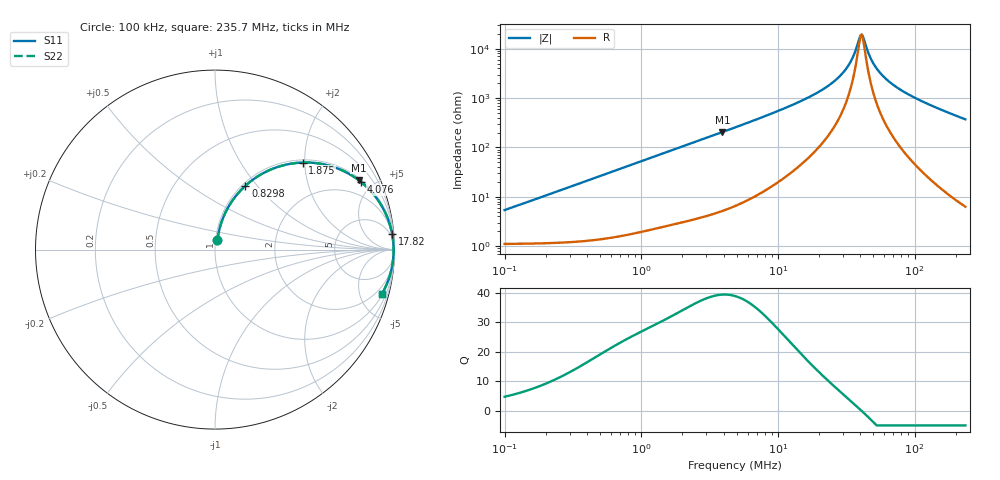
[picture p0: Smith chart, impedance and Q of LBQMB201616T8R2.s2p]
! LBQMB201616T8R2  S-PARAMETER MODEL  ( General Type )
! Model Generated by TAIYO YUDEN Corporation (http://www.ty-top.com)
! Version 1.0
! TAIYO YUDEN Control No. 191025NI43SB-FBB
! Copyright(c) 2019 TAIYO YUDEN CO.,LTD. All Rights Reserved.
! Product Description (link to TY-COMPAS)
! https://ds.yuden.co.jp/TYCOMPAS/or/detail?pn=LBQMB201616T8R2J&u=M
! Products Name : Inductors
! Characteristics :
!  Inductance : 8.2 uH , SRF(min) : 30 MHz , DC Resistance(max) : 1.43 Ohm , Rated Current : 225 mA
!  Case Size : 2.0 x 1.6 / 0.079 x 0.063 [mm/inch] , Thickness : 1.6 / 0.063 [mm/inch]
!  (Conditions: Temperature = 25 degC , DC Bias Current/Voltage = 0A / 0V)
! External Node Assignments :
!  1  o---GGG---o  2
! GND o---------o GND
! Frequency Range : 0.1MHz  -  235.669543MHz  [ 402 STEP ]
# MHz S RI R 50
! Freq[MHz].  S11 Real  S11 Imag  S21 Real  S21 Imag  S12 Real  S12 Imag  S22 Real  S22 Imag
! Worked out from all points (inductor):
!   401 points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, 100 kHz to 235.7 MHz, reference 50 ohm
!   read as one part in series: L = 8.41 uH near 104 kHz
!   highest Q = 39.5 at 3.921 MHz (marker M1), where L = 8.28 uH
!   self-resonance near 40.28 MHz
!   S11 on the Smith chart (normalised r, x): 100 kHz: 1.02, +0.11; 829.8 kHz: 1.03, +0.87; 1.875 MHz: 1.06, +1.95; 4.076 MHz: 1.11, +4.24; 17.82 MHz: 2, +23; 235.7 MHz: 1.13, -7.42
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0.1  0.0137 0.0516  0.9863 -0.0516  0.9863 -0.0516  0.0137 0.0516
0.367165  0.0473 0.1823  0.9527 -0.1823  0.9527 -0.1823  0.0473 0.1823
0.82976  0.1694 0.3556  0.8306 -0.3556  0.8306 -0.3556  0.1694 0.3556
1.348099  0.3365 0.4561  0.6635 -0.4561  0.6635 -0.4561  0.3365 0.4561
1.875187  0.4881 0.4851  0.5119 -0.4851  0.5119 -0.4851  0.4881 0.4851
3.921149  0.8004 0.3872  0.1996 -0.3872  0.1996 -0.3872  0.8004 0.3872
4.076382  0.8123 0.378  0.1877 -0.378  0.1877 -0.378  0.8123 0.378
4.854581  0.8592 0.3352  0.1408 -0.3352  0.1408 -0.3352  0.8592 0.3352
10.15127  0.9628 0.1719  0.0372 -0.1719  0.0372 -0.1719  0.9628 0.1719
17.8243  0.9867 0.0868  0.0133 -0.0868  0.0133 -0.0868  0.9867 0.0868
24.3167  0.9919 0.0511  0.0081 -0.0511  0.0081 -0.0511  0.9919 0.0511
30.10531  0.9938 0.0293  0.00619 -0.0293  0.00619 -0.0293  0.9938 0.0293
34.48723  0.9945 0.0162  0.0055 -0.0162  0.0055 -0.0162  0.9945 0.0162
39.50697  0.9949 0.0033  0.00515 -0.0033  0.00515 -0.0033  0.9949 0.0033
41.07099  0.9949 -0.000367  0.00511 0.000367  0.00511 0.000367  0.9949 -0.000367
42.69694  0.9949 -0.00404  0.0051 0.00404  0.0051 0.00404  0.9949 -0.00404
47.04901  0.9948 -0.0133  0.00518 0.0133  0.00518 0.0133  0.9948 -0.0133
50.84796  0.9946 -0.0207  0.00537 0.0207  0.00537 0.0207  0.9946 -0.0207
57.12919  0.9941 -0.0322  0.00589 0.0322  0.00589 0.0322  0.9941 -0.0322
65.44454  0.9931 -0.0461  0.00687 0.0461  0.00687 0.0461  0.9931 -0.0461
106.3267  0.9846 -0.1043  0.0154 0.1043  0.0154 0.1043  0.9846 -0.1043
235.6695  0.9286 -0.2491  0.0714 0.2491  0.0714 0.2491  0.9286 -0.2491
